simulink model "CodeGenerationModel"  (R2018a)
settings: Solver=FixedStepDiscrete  StartTime=0.0  StopTime=Inf  RelTol=1e-3  EnableMultiTasking=on
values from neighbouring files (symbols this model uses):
  Anglog_Input_Max = 3    [ParameterInitializationFileFinal.m]    (also in Panda_BEVintage_VPE_S_Data_CodeGen_Model.m = 10; Panda_BEVintage_VPE_S_Data_Enhanced_Model.m = 10)
  Anglog_Input_Min = 0    [ParameterInitializationFileFinal.m]    (also in Panda_BEVintage_VPE_S_Data_CodeGen_Model.m = -10; Panda_BEVintage_VPE_S_Data_Enhanced_Model.m = -10)
  Bits = 12    [ParameterInitializationFileFinal.m]    (also in Panda_BEVintage_VPE_S_Data_CodeGen_Model.m = 16; Panda_BEVintage_VPE_S_Data_Enhanced_Model.m = 16)
  Frequency_Signal = 1/2    (= 0.5)    [ParameterInitializationFileFinal.m]
  Max_Signal = Amplitude_Signal+Bias_Signal    (= 5)    [ParameterInitializationFileFinal.m]
  Min_Signal = -Amplitude_Signal+Bias_Signal    (= -5)    [ParameterInitializationFileFinal.m]
undefined symbols (not defined in the file or in its folder): ADCINA0, ADCINA1, ADCINA2, ADCINA3, ADCINA4, ADCINA5, ADCINA6, ADCINA7, ADCINB0, ADCINB1, ADCINB2, ADCINB3, ADCINB4, ADCINB5, ADCINB6, ADCINB7
libraries: c280xlib x2, dspfdesign x2, c2833xlib x1

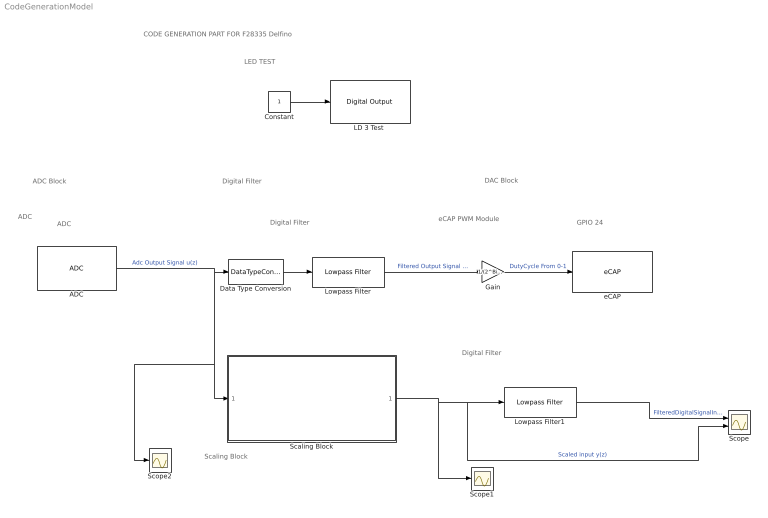
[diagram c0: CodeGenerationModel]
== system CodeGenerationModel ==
  note: GPIO 24
  note: LED TEST
  note: eCAP PWM Module
  note: Digital Filter
  note: CODE GENERATION PART FOR F28335 Delfino
  note: ADC
  note: ADC
  note: ADC Block
  note: DAC Block
  note: Scaling Block
  note: Digital Filter
  note: Digital Filter
  ADC : c280xlib/ADC  useModule=A  useMode=Sequential  sourceSOC=Software  sourceSOC1=Software  sourceSOC2=ePWMxB  xint2_ADCSOC=31  Ts=0.01  dType=uint16  postInterrupt=off  numConversionsSingle=1  numConversionsDouble=1  conv0=ADCINA0  conv1=ADCINA1  conv2=ADCINA2  conv3=ADCINA3  conv4=ADCINA4  conv5=ADCINA5  conv6=ADCINA6  conv7=ADCINA7  conv8=ADCINB0  conv9=ADCINB1  conv10=ADCINB2  conv11=ADCINB3  conv12=ADCINB4  conv13=ADCINB5  conv14=ADCINB6  conv15=ADCINB7  convAB0=ADCINA0 and ADCINB0  convAB1=ADCINA1 and ADCINB1  convAB2=ADCINA2 and ADCINB2  convAB3=ADCINA3 and ADCINB3  convAB4=ADCINA4 and ADCINB4  convAB5=ADCINA5 and ADCINB5  convAB6=ADCINA6 and ADCINB6  convAB7=ADCINA7 and ADCINB7  convA0=ADCINA0  convA1=ADCINA0  convA2=ADCINA2  convA3=ADCINA3  convA4=ADCINA4  convA5=ADCINA5  convA6=ADCINA6  convA7=ADCINA7  convB0=ADCINB0  convB1=ADCINB1  convB2=ADCINB2  convB3=ADCINB3  convB4=ADCINB4  convB5=ADCINB5  convB6=ADCINB6  convB7=ADCINB7  c28xmultiPort=off  endma=off  chdma=1
  Constant : Constant  SampleTime=2
  Data Type Conversion : DataTypeConversion
  Gain : Gain  Gain=1/(2^Bits -1) *100
  "LD 3 Test " : c2833xlib/Digital Output  GPIO_Number=GPIO32~GPIO39  GPIO_Bit0=off  GPIO_BIT0_Toggle=off  GPIO_Bit1=off  GPIO_BIT1_Toggle=off  GPIO_Bit2=on  GPIO_BIT2_Toggle=on  GPIO_Bit3=off  GPIO_BIT3_Toggle=off  GPIO_Bit4=off  GPIO_BIT4_Toggle=off  GPIO_Bit5=off  GPIO_BIT5_Toggle=off  GPIO_Bit6=off  GPIO_BIT6_Toggle=off  GPIO_Bit7=off  GPIO_BIT7_Toggle=on
  Lowpass Filter : dspfdesign/Lowpass Filter  FilterType=IIR  DesignForMinimumOrder=off  FilterOrder=1  PassbandFrequency=Frequency_Signal*4  StopbandFrequency=1  PassbandRipple=1  StopbandAttenuation=80  InheritSampleRate=on  SampleRate=Frequency_Signal*9  SimulateUsing=Interpreted execution  roundingMode=Floor  coeffsDataTypeStr=fixdt(1,16)
  Lowpass Filter1 : dspfdesign/Lowpass Filter  FilterType=IIR  DesignForMinimumOrder=off  FilterOrder=1  PassbandFrequency=Frequency_Signal*4  StopbandFrequency=1  PassbandRipple=1  StopbandAttenuation=80  InheritSampleRate=on  SampleRate=Frequency_Signal*9  SimulateUsing=Interpreted execution  roundingMode=Floor  coeffsDataTypeStr=fixdt(1,16)
  Scaling Block : Subsystem
  Scope : Scope  NumInputPorts=2
  Scope1 : Scope
  Scope2 : Scope
  eCAP : c280xlib/eCAP  operatingMode=APWM  selectCAPx=eCAP1  offsetValue=0  counterSynIn=off  enableCounter=off  syncOutput=CTR=PRD  sampleTime=0.001  eventPrescaler=0  selectMode=Continuous  enableOneShot=off  stopValue=Capture Event 1  resetEv1Ts=off  ev1Polarity=Rising Edge  resetEv2Ts=off  ev2Polarity=Rising Edge  resetEv3Ts=off  ev3Polarity=Rising Edge  resetEv4Ts=off  ev4Polarity=Rising Edge  tSCntrDataType=uint32  capEvFlag=off  capFlagDataType=uint16  overFlowFlag=off  overFlowFlagDataType=uint16  periodUnit=Seconds  periodSource=Specify via dialog  waveformPeriod=tpwm  dutyUnit=Percentages  dutySource=Input port  dutyCycle=50  outputPolarity=Active High  enableCEVT1Int=off  enableCEVT2Int=off  enableCEVT3Int=off  enableCEVT4Int=off  enableCTROVFInt=off  enablePRDInt=off  enableCMPInt=off
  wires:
  Constant/1 -> "LD 3 Test "/1
  ADC/1 -> Data Type Conversion/1, Scope2/1, Scaling Block/1(u(z))  "Adc Output Signal u(z)"
  Gain/1 -> eCAP/1  "DutyCycle From 0-1"
  Lowpass Filter/1 -> Gain/1  "Filtered Output Signal dy(z)"
  Scaling Block/1(Scaled input y(z)) -> Scope/2, Lowpass Filter1/1, Scope1/1  "Scaled input y(z)"
  Lowpass Filter1/1 -> Scope/1  "FilteredDigitalSignalInReferenceValue yz(z)"
  Data Type Conversion/1 -> Lowpass Filter/1

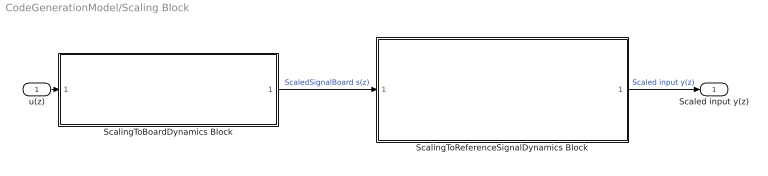
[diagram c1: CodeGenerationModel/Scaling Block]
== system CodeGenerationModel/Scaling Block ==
  u(z) : Inport
  ScalingToBoardDynamics Block : Subsystem
  ScalingToReferenceSignalDynamics Block : Subsystem
  Scaled input y(z) : Outport
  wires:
  ScalingToBoardDynamics Block/1(ScaledToBoardValues) -> ScalingToReferenceSignalDynamics Block/1(ScaledToBoardValues)  "ScaledSignalBoard s(z)"
  u(z)/1 -> ScalingToBoardDynamics Block/1(DigitalSignalFromAnalogPinA0)
  ScalingToReferenceSignalDynamics Block/1("ScaledInReferenceSignalDynamics ") -> Scaled input y(z)/1  "Scaled input y(z)"

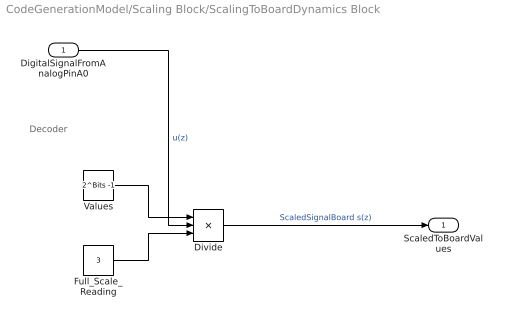
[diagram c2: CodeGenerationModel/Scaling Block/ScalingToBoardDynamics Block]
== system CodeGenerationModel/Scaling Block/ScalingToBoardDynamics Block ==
  note: Decoder
  DigitalSignalFromAnalogPinA0 : Inport
  Divide : Product  Inputs=/**
  Full_Scale_Reading : Constant  Value=3
  Values : Constant  Value=2^Bits -1
  ScaledToBoardValues : Outport
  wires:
  DigitalSignalFromAnalogPinA0/1 -> Divide/2  "u(z)"
  Values/1 -> Divide/1
  Divide/1 -> ScaledToBoardValues/1  "ScaledSignalBoard s(z)"
  Full_Scale_Reading/1 -> Divide/3

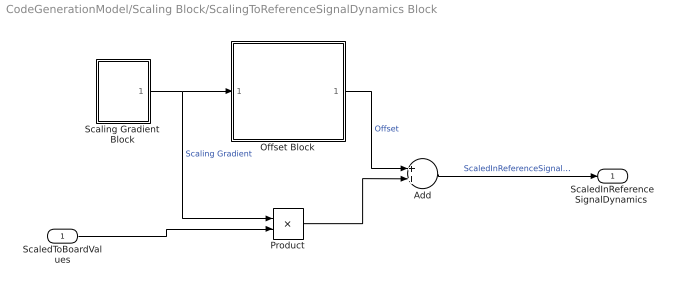
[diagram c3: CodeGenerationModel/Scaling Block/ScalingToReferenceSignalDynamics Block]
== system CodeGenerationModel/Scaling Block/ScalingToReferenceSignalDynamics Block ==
  ScaledToBoardValues : Inport
  Add : Sum
  Offset Block : Subsystem
  Product : Product
  Scaling Gradient Block : Subsystem
  "ScaledInReferenceSignalDynamics " : Outport
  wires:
  ScaledToBoardValues/1 -> Product/2
  Product/1 -> Add/2
  Scaling Gradient Block/1("Gradient ") -> Product/1, Offset Block/1("Gradient ")  "Scaling Gradient"
  Offset Block/1("Offset ") -> Add/1  "Offset"
  Add/1 -> "ScaledInReferenceSignalDynamics "/1  "ScaledInReferenceSignalDynamics y(z)"

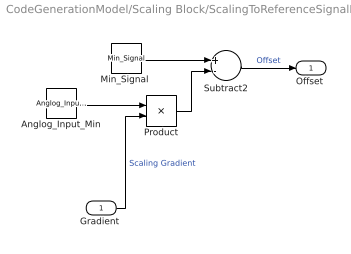
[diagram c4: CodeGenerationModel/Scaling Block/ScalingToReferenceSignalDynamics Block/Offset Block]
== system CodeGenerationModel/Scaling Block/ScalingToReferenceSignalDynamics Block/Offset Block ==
  "Gradient " : Inport
  Anglog_Input_Min : Constant  Value=Anglog_Input_Min
  "Min_Signal " : Constant  Value=Min_Signal
  Product : Product
  Subtract2 : Sum  Inputs=+-
  "Offset " : Outport
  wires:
  Anglog_Input_Min/1 -> Product/1
  "Gradient "/1 -> Product/2  "Scaling Gradient"
  Product/1 -> Subtract2/2
  Subtract2/1 -> "Offset "/1  "Offset"
  "Min_Signal "/1 -> Subtract2/1

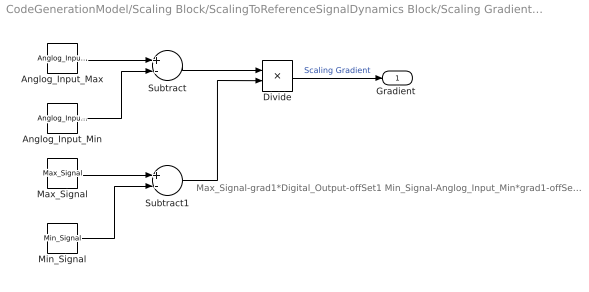
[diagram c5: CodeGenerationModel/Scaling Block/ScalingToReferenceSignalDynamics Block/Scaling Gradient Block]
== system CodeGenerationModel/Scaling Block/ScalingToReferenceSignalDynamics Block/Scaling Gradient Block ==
  note: Max_Signal-grad1*Digital_Output-offSet1 Min_Signal-Anglog_Input_Min*grad1-offSet1
  Anglog_Input_Max : Constant  Value=Anglog_Input_Max
  Anglog_Input_Min : Constant  Value=Anglog_Input_Min
  Divide : Product  Inputs=/*
  Max_Signal : Constant  Value=Max_Signal
  Min_Signal : Constant  Value=Min_Signal
  Subtract : Sum  Inputs=+-
  Subtract1 : Sum  Inputs=+-
  "Gradient " : Outport
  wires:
  Divide/1 -> "Gradient "/1  "Scaling Gradient"
  Subtract1/1 -> Divide/2
  Subtract/1 -> Divide/1
  Anglog_Input_Min/1 -> Subtract/2
  Min_Signal/1 -> Subtract1/2
  Max_Signal/1 -> Subtract1/1
  Anglog_Input_Max/1 -> Subtract/1
